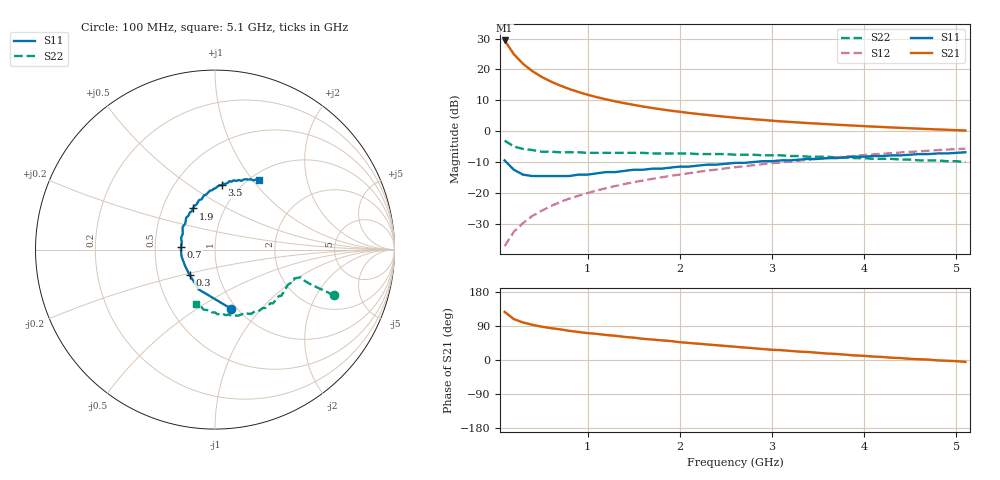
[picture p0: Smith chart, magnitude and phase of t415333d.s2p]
!AT-41533
!S and NOISE PARAMETERS at Vce=2.7V Ic=25mA. LAST UPDATED 01-25-95
# ghz s ma r 50
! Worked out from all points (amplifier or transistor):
!   51 points, 100 MHz to 5.1 GHz, reference 50 ohm
!   highest |S21| = 29.4 dB at 100 MHz (marker M1)
!   |S21| within 3 dB of that: start of sweep to 167.7 MHz
!   unconditionally stable (mu >= 1): 376.7 MHz to 2.244 GHz
!   at 900 MHz: K = 1.07, MAG = 15.2 dB, |S12| = -20.8 dB
!   at 2.6 GHz: K = 0.97, MSG = 8.0 dB, |S12| = -11.6 dB
!   at 5.1 GHz: K = 0.88, MSG = 2.9 dB, |S12| = -5.6 dB
!   lowest NFmin = 1.30 dB at 100 MHz
!   S11 on the Smith chart (normalised r, x): 100 MHz: 0.94, -0.70; 300 MHz: 0.73, -0.21; 700 MHz: 0.68, +0.02; 1.9 GHz: 0.71, +0.35; 3.5 GHz: 0.83, +0.68; 5.1 GHz: 1.09, +1.08
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0.1  0.34 -75.0  29.4 127.0  0.014 72.0  0.71 -21.0
0.2  0.24 -112.0  17.65 108.0  0.024 73.0  0.57 -20.0
0.3  0.2 -135.0  12.32 99.0  0.033 75.0  0.52 -19.0
0.4  0.19 -151.0  9.418 93.0  0.043 76.0  0.5 -18.0
0.5  0.19 -168.0  7.614 88.0  0.052 76.0  0.47 -20.0
0.6  0.19 -179.0  6.4 84.0  0.062 76.0  0.47 -21.0
0.7  0.19 175.0  5.517 81.0  0.072 76.0  0.46 -22.0
0.8  0.19 167.0  4.845 77.0  0.082 75.0  0.46 -23.0
0.9  0.2 161.0  4.329 74.0  0.091 74.0  0.46 -24.0
1  0.2 154.0  3.909 71.0  0.101 74.0  0.45 -26.0
1.1  0.21 149.0  3.568 69.0  0.111 73.0  0.45 -27.0
1.2  0.22 145.0  3.294 66.0  0.121 72.0  0.45 -29.0
1.4  0.23 135.0  2.854 61.0  0.141 71.0  0.45 -32.0
1.6  0.24 128.0  2.522 56.0  0.161 69.0  0.45 -35.0
1.8  0.25 121.0  2.271 52.0  0.181 67.0  0.44 -38.0
1.9  0.26 118.0  2.163 50.0  0.191 66.0  0.44 -39.0
2.2  0.28 110.0  1.91 43.0  0.222 63.0  0.43 -44.0
2.6  0.31 101.0  1.667 35.0  0.263 59.0  0.42 -51.0
3  0.33 93.0  1.489 27.0  0.305 54.0  0.41 -59.0
3.5  0.36 84.0  1.333 19.0  0.36 48.0  0.39 -69.0
4.3  0.41 71.0  1.157 6.0  0.446 38.0  0.36 -88.0
5.1  0.46 58.0  1.032 -5.0  0.527 28.0  0.32 -109.0
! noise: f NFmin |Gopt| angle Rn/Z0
0.1  1.3  0.1  24  0.12
0.9  1.6  0.25  -158  0.11
1.8  1.9  0.48  -122  0.19
2.4  2.1  0.59  -101  0.37
